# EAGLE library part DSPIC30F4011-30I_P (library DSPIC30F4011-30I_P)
Digital Signal Controllers Source: Datasheet
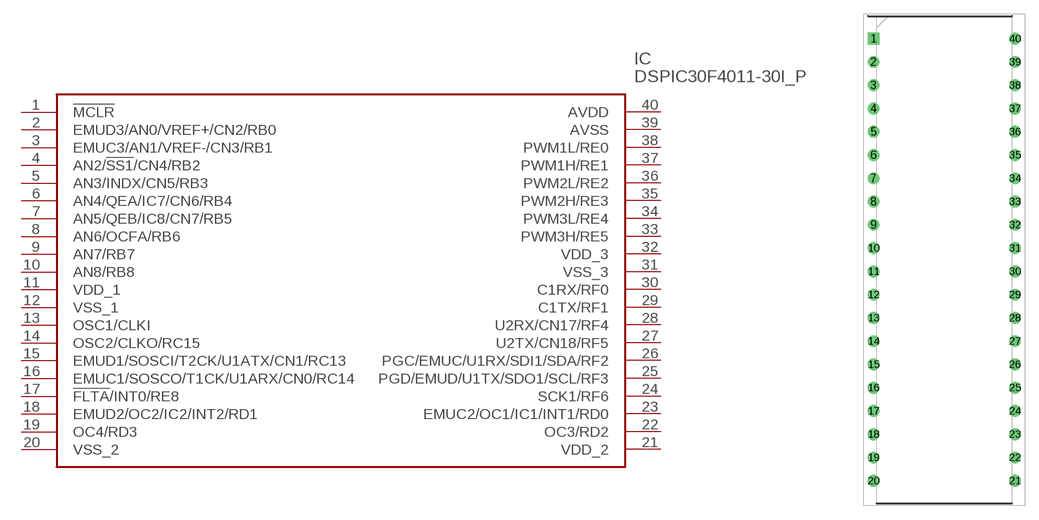
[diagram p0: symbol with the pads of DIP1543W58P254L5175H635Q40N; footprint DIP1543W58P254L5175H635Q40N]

Designator prefix IC

## DSPIC30F4011-30I_P (Arrow_Part_Number: dsPIC30F4011-30I/P; Arrow_Price-Stock: https://www.arrow.com/en/products/dspic30f4011-30ip/microchip-technology; Description: Digital Signal Controllers; Height: 6.35mm; Manufacturer_Name: Microchip; Manufacturer_Part_Number: DSPIC30F4011-30I/P; Mouser_Part_Number: 579-30F4011-30I/P; Mouser_Price-Stock: https://www.mouser.co.uk/ProductDetail/Microchip-Technology/dsPIC30F4011-30I-P?qs=nMCt4TBfEwpnzUUd8LIZNg%3D%3D)  [DIP1543W58P254L5175H635Q40N]
1  !MCLR
2  EMUD3/AN0/VREF+/CN2/RB0
3  EMUC3/AN1/VREF-/CN3/RB1
4  AN2/!SS1!/CN4/RB2
5  AN3/INDX/CN5/RB3
6  AN4/QEA/IC7/CN6/RB4
7  AN5/QEB/IC8/CN7/RB5
8  AN6/OCFA/RB6
9  AN7/RB7
10  AN8/RB8
11  VDD_1
12  VSS_1
13  OSC1/CLKI
14  OSC2/CLKO/RC15
15  EMUD1/SOSCI/T2CK/U1ATX/CN1/RC13
16  EMUC1/SOSCO/T1CK/U1ARX/CN0/RC14
17  !FLTA!/INT0/RE8
18  EMUD2/OC2/IC2/INT2/RD1
19  OC4/RD3
20  VSS_2
21  VDD_2
22  OC3/RD2
23  EMUC2/OC1/IC1/INT1/RD0
24  SCK1/RF6
25  PGD/EMUD/U1TX/SDO1/SCL/RF3
26  PGC/EMUC/U1RX/SDI1/SDA/RF2
27  U2TX/CN18/RF5
28  U2RX/CN17/RF4
29  C1TX/RF1
30  C1RX/RF0
31  VSS_3
32  VDD_3
33  PWM3H/RE5
34  PWM3L/RE4
35  PWM2H/RE3
36  PWM2L/RE2
37  PWM1H/RE1
38  PWM1L/RE0
39  AVSS
40  AVDD

## Footprint DIP1543W58P254L5175H635Q40N (pad centres in mm)
40 ld PDIP (P) 600 mil
drill 0.784 pad 1.184 square: 1 -7.715,24.13
drill 0.784 pad 1.184: 2 -7.715,21.59; 3 -7.715,19.05; 4 -7.715,16.51; 5 -7.715,13.97; 6 -7.715,11.43; 7 -7.715,8.89; 8 -7.715,6.35; 9 -7.715,3.81; 10 -7.715,1.27; 11 -7.715,-1.27; 12 -7.715,-3.81; 13 -7.715,-6.35; 14 -7.715,-8.89; 15 -7.715,-11.43; 16 -7.715,-13.97; 17 -7.715,-16.51; 18 -7.715,-19.05; 19 -7.715,-21.59; 20 -7.715,-24.13; 21 7.715,-24.13; 22 7.715,-21.59; 23 7.715,-19.05; 24 7.715,-16.51; 25 7.715,-13.97; 26 7.715,-11.43; 27 7.715,-8.89; 28 7.715,-6.35; 29 7.715,-3.81; 30 7.715,-1.27; 31 7.715,1.27; 32 7.715,3.81; 33 7.715,6.35; 34 7.715,8.89; 35 7.715,11.43; 36 7.715,13.97; 37 7.715,16.51; 38 7.715,19.05; 39 7.715,21.59; 40 7.715,24.13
